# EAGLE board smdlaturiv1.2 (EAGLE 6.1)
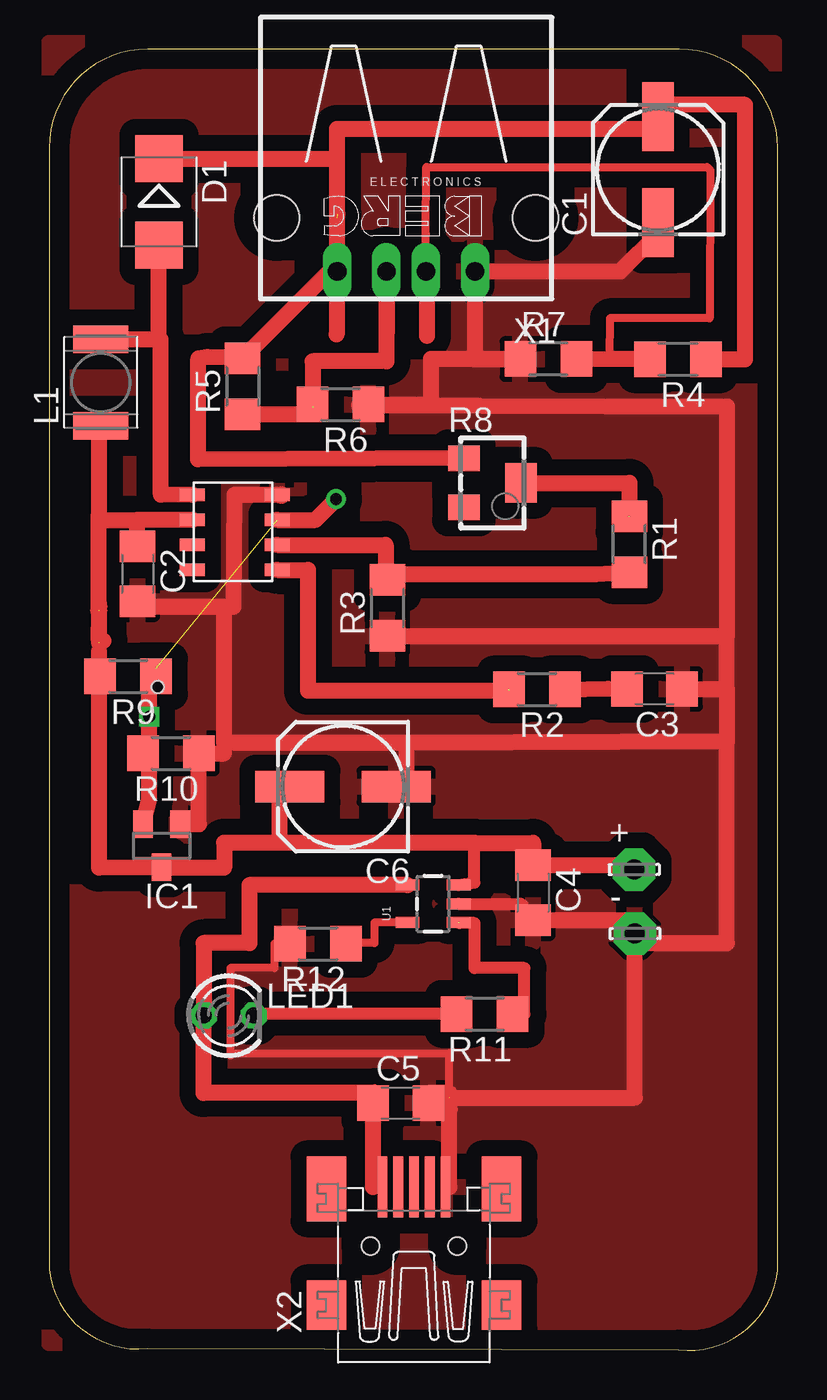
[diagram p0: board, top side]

Size 37 x 66.11 mm. Coordinates in mm from the lower left corner, seen from the top.
Outline: 32,66.11 5,66.11 arc90 0,61.11 0,4.1 arc90 4.99,0.1 31.99,0.03 arc90 37,4.03 37,61.11 arc90 32,66.11
Copper layers (1*16): Top 0.035mm / dielectric 1.5mm / Bottom 0.035mm
Design rules: minimum track width 10mil, minimum drill 24mil, track to track 8mil, track to pad 8mil, pad to pad 8mil, via to via 8mil, smd to smd 8mil, copper to edge 40mil, drill to drill 8mil, minimum pad ring 10mil, minimum via ring 8mil, stop-mask expansion 4mil, vias tented up to drill 0mil, thermal gap 10mil
Holes 0.6 mm at 5.52,33.7

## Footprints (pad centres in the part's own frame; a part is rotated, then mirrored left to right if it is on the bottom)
LSP10 = drill 1.016 pad 2.159 octagon: MP 0,0
153CLV-0605 = smd 3.5 x 1.6: + 2.7,0; - -2.7,0
C1206 = smd 1.6 x 1.8: 1 -1.4,0; 2 1.4,0
SMB = smd 2.4 x 2.4: A 2.2,0; C -2.2,0
SOT23 = smd 1 x 1.4: 1 -0.95,-1.1; 2 0.95,-1.1; 3 0,1.1
L5038P = smd 1.4 x 2.8: 1 -2.2,0; 2 2.2,0
LED3MM = drill 0.813 octagon: A -1.27,0; K 1.27,0
R1206 = smd 1.6 x 1.803: 1 -1.422,0; 2 1.422,0
RTRIM3224W = smd 1.3 x 1.6: 1 -1.25,-1.45; 3 1.25,-1.45 | smd 2 x 1.6: 2 0,1.45
SOT23-5 = smd 0.55 x 1.2: 1 -0.95,-1.3; 2 0,-1.3; 3 0.95,-1.3; 4 0.95,1.3; 5 -0.95,1.3
LT1308 = smd 1.27 x 0.635: 1 -0.25,4.445; 2 -0.25,3.175; 3 -0.25,1.905; 4 -0.25,0.635; 5 4.06,0.635; 6 4.06,1.905; 7 4.06,3.175; 8 4.06,4.445
PN87520 = drill 0.95 long: 1 -3.5,2.71; 2 -1,2.71; 3 1,2.71; 4 3.5,2.71 | hole 2.3: -6.57,0; 6.57,0
32005-301 = smd 3.1 x 0.5: 1 3,1.6; 2 3,0.8; 3 3,0; 4 3,-0.8; 5 3,-1.6 | smd 2.5 x 2: M1 -3,-4.45; M2 -3,4.45 | smd 3.3 x 2: M3 2.9,4.45; M4 2.9,-4.45 | hole 0.9: 0,2.2; 0,-2.2

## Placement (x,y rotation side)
+  LSP10  [LSP10]  29.71,24.43 0 top
-  LSP10  [LSP10]  29.74,21.17 0 top
C1  100uf  [153CLV-0605]  30.93,59.99 90 top
C2  10uf  [C1206]  4.49,39.46 270 top
C3  22nf  [C1206]  30.75,33.6 180 top
C4  4.7uf  [C1206]  24.57,23.26 270 top
C5  4.7uf  [C1206]  17.85,12.57 0 top
C6  100uf  [153CLV-0605]  14.92,28.64 180 top
D1  scotty  [SMB]  5.57,58.35 270 top
IC1  TCM810  [SOT23]  5.71,25.64 180 top
L1  4.7uh  [L5038P]  2.62,49.17 90 top
LED1  [LED3MM]  9.11,17.01 0 top
R1  301k  [R1206]  29.46,40.95 270 top
R2  47k  [R1206]  24.76,33.58 180 top
R3  100k  [R1206]  17.17,37.72 90 top
R4  75k  [R1206]  31.93,50.35 180 top
R5  75k  [R1206]  9.82,48.98 90 top
R6  49.9k  [R1206]  14.79,48.05 180 top
R7  49.9k  [R1206]  25.35,50.37 0 top
R8  [RTRIM3224W]  22.51,44.07 270 top
R9  100k  [R1206]  4.01,34.24 180 top
R10  100k  [R1206]  6.18,30.33 180 top
R11  470  [R1206]  22.12,17.09 180 top
R12  2k  [R1206]  13.65,20.66 180 top
U1  MCP73831  [SOT23-5]  19.5,22.69 90 top
U$1  LT1308  [LT1308]  11.33,44.1 180 top
X1  [PN87520]  18.13,57.53 180 top
X2  MINI-USB-32005-301  [32005-301]  18.53,5.3 90 top

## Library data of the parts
+ - = solpad
C1-C6 L1 R1-R12 = resistor
D1 = diode
IC1 = maxim; MF: MAXIM; MPN: MAX6520EUR-T; OC_FARNELL: unknown; OC_NEWARK: 02J4586
LED1 = led
U1 = SparkFun-PowerIC
U$1 = lt1308
X1 = con-berg; OC_FARNELL: unknown; OC_NEWARK: unknown
X2 = con-cypressindustries; OC_FARNELL: unknown; OC_NEWARK: unknown

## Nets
+5V: D1.C R4.1 R5.2 R8.1 X1.4
GND: -.MP C2.2 C3.1 C4.2 C5.2 C6.- IC1.1 R3.1 R6.1 R7.1 R10.1 R12.2 U1.2 U$1.4 X1.1 X2.5
N$1: R1.2 R3.2 U$1.2
N$2: R2.2 U$1.1
N$4: C3.2 R2.1
N$5: D1.A L1.2 U$1.5
N$6: R4.2 R7.2 X1.2
N$7: R5.1 R6.2 X1.3
N$11: IC1.2 R9.1 R10.2 U$1.3
N$13: R1.1 R8.2
N$14: C5.1 LED1.A U1.4 X2.1
N$16: LED1.K R11.2
N$17: R11.1 U1.1
N$19: R12.1 U1.5
V+: +.MP C2.1 C4.1 C6.+ IC1.3 L1.1 R9.2 U1.3 U$1.6

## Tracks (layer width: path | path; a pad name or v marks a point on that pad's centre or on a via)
+5V  (1 unrouted)
  Top 0.813: R4.1 35.34,50.36 35.34,63.28 30.93,63.28 30.93,63.24 30.92,63.23 30.92,62.05 | X1.4 14.66,54.82 | 7.57,45.61 7.57,45.66 | 7.57,45.66 7.57,50.39 8.03,50.47 R5.2 14.24,54.82 X1.4 | X1.4 14.63,57.74 | 30.92,62.05 30.93,62.05 | D1.C 14.61,60.55 | 14.61,60.55 14.61,57.53 | 30.92,62.05 14.61,62.05 14.61,60.55 | R8.1 7.57,45.26 7.57,45.66
GND  (2 unrouted)
  Top 0.406: 8.89,30.33 8.89,30.86 | C4.2 23.94,22.69 24.13,22.69 24.13,21.97 | 29.3,20.7 -.MP | X2.5 20.32,8.3 | 19.25,13.08 C5.2 | 9.22,15.09 20.3,15.09 20.3,12.31 | R12.2 11.43,20.66 11.43,19.43 9.21,19.43 9.21,14.98
  Top 0.61: U1.2 23.94,22.69
  Top 0.813: R6.1 18.81,48.05 | 18.81,48.05 18.83,48.03 | 18.83,48.03 18.81,48.02 | 11.8,43.46 11.8,43.48 | 11.8,43.46 U$1.4 9.4,43.46 9.35,37.77 8.89,37.77 | 11.8,43.46 11.8,43.41 | 18.85,48.06 18.83,48.03 | 8.89,37.77 4.44,37.77 C2.2 | 18.81,48.05 19.4,48.05 19.4,50.37 R7.1 21.61,50.34 21.61,54.82 X1.1 29.01,54.82 30.93,56.74 | IC1.1 7.6,26.74 R10.1 8.89,30.33 | 8.89,37.77 8.89,30.86 18.16,30.86 | C4.2 29.3,21.86 -.MP | 34.42,30.92 18.16,30.86 | 29.3,20.7 34.42,20.7 34.42,30.92 | 34.42,36.3 34.42,47.95 15.72,48.01 | 34.42,33.6 34.42,30.92 | C6.- 18.16,28.64 18.16,30.86 | R3.1 34.42,36.3 | C3.1 34.42,33.6 | 34.42,33.6 34.42,36.3 | 20.32,8.3 20.32,13.08 19.25,13.08 | 20.33,12.84 29.75,12.84 29.75,21.13 | 20.3,12.31 20.34,12.31 | 20.34,12.31 20.34,12.84 | 20.34,12.31 20.34,12.2
  pour Top (isolate 0.813): 0,61.34 0,0.38 36.83,0.38 36.83,66.42 0,66.42
N$1
  Top 0.813: U$1.2 17.08,40.92 17.08,39.43 | 17.08,39.14 17.08,38.92 | R3.2 17.08,39.14 | 17.08,39.14 17.08,39.43 | 17.08,39.43 27.75,39.43 R1.2
N$2  (1 unrouted)
  Top 0.813: U$1.1 13.14,39.65 13.14,38.42 13.13,33.52 23.38,33.52
N$4
  Top 0.813: R2.1 28.37,33.61 C3.2
N$5
  Top 0.813: L1.2 5.65,51.37 | 5.65,51.37 5.57,51.37 D1.A | U$1.5 5.67,43.48 5.65,51.37
N$6
  Top 0.406: 19.09,54.82 X1.2 19.13,56.73 19.16,60.12 33.41,60.12 33.58,59.95 33.55,52.43 28.47,52.43 28.45,50.39
  Top 0.813: R7.2 28.45,50.39 30.51,50.39 R4.2
N$7  (1 unrouted)
  Top 0.813: R5.1 13.67,47.57 13.67,48.07 13.68,48.07 | 13.68,48.07 13.75,48.07 | X1.3 17.12,51.7 17.12,50.25 13.38,50.25 13.38,47.93 | 13.68,48.07 R6.2 13.38,47.95
N$8  (via drill 0.6)
  other vias: 14.57,43.25
N$11  (via drill 0.6)  (1 unrouted)
  Top 0.406: 5.08,34.67 5.43,34.67 R9.1 | R10.2 5.08,31.6
  Top 0.813: U$1.3 13.51,42.19 14.53,43.2 | IC1.2 5.08,28.01 5.08,31.6 v5.08,32.19 5.08,34.67
N$13  (1 unrouted)
  Top 0.813: R8.2 29.46,44.07 29.46,42.35
N$14
  Top 0.406: X2.1 16.45,8.3 | C5.1 16.51,13.33 16.51,13.08
  Top 0.813: 16.45,8.3 C5.1 | 16.51,13.08 7.84,13.08 LED1.A 7.84,20.7 10.16,20.7 10.16,23.64 U1.4
N$16
  Top 0.406: 10.38,17.09 LED1.K
  Top 0.61: R11.2 10.38,17.09
N$17  (1 unrouted)
  Top 0.406: R11.1 24.13,17.09
  Top 0.61: 24.13,17.09 24.13,19.43 21.59,19.43 21.59,21.72 20.83,21.72
N$19
  Top 0.406: U1.5 16.51,21.74 16.51,20.7 15.07,20.7 R12.1
S$4
  Top 0.813: 19.14,54.7 19.18,54.7 19.18,51.54
S$5
  Top 0.813: 17.09,54.66 17.13,54.66 17.13,51.67
S$6
  Top 0.813: 14.74,54.62 14.59,54.62 14.59,51.62
V+  (2 unrouted)
  Top 0.406: C2.1 4.5,40.86 | R9.2 2.54,35.51 2.54,35.94 | 5.71,24.51 IC1.3
  Top 0.61: U1.3 21.59,23.76 21.59,25.78
  Top 0.813: L1.1 2.53,46.97 2.53,42.19 | U$1.6 4.48,42.19 | 2.52,42.19 2.52,37.61 | 2.52,42.19 2.52,42.49 | 2.53,42.19 2.52,42.19 | 2.52,37.61 2.52,36.73 | 2.52,36.28 2.52,36.07 2.52,35.94 | 2.52,36.28 2.52,36.73 | 2.52,37.43 2.51,36.67 2.52,36.73 | 2.53,37.25 2.52,37.92 2.53,37.7 2.52,37.55 2.51,37.52 2.5,37.7 | 2.52,37.61 2.52,36.29 | 4.5,40.86 4.48,40.86 4.48,42.19 | 2.53,42.19 4.48,42.19 | 2.75,36.05 2.52,36.28 | IC1.3 2.54,24.52 2.54,35.51 | +.MP 29.71,24.66 C4.1 24.57,25.78 21.59,25.78 11.54,25.78 | 11.54,25.78 8.89,25.78 8.89,24.51 5.71,24.51 | C6.+ 11.68,28.64 11.68,25.84 11.54,25.84 11.54,25.78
